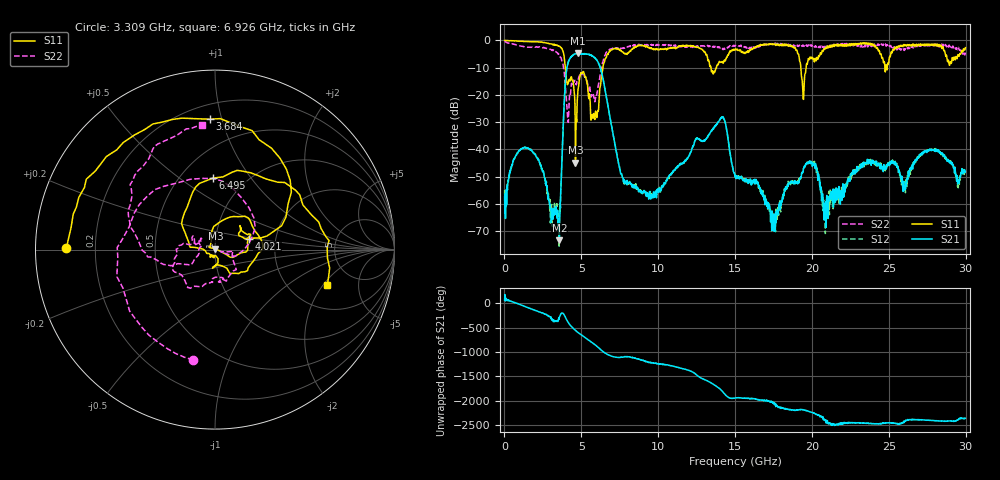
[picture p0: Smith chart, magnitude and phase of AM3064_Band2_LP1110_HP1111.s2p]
# Hz S DB R 50.0
!freq dBS11 angS11 dBS21 angS21 dBS12 angS12 dBS22 angS22
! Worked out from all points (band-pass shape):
!   1600 points, 10 MHz to 29.98 GHz, reference 50 ohm
!   highest |S21| = -4.74 dB at 4.752 GHz (marker M1); lowest = -73.2 dB at 3.571 GHz (marker M2)
!   |S21| within 3 dB of the highest: 4.171 GHz to 6.062 GHz (1.89 GHz wide, 36.9 % of centre)
!   lowest |S11| = -44.8 dB at 4.621 GHz (marker M3), VSWR 1.01, Z = 50.3 + j0.512 ohm
!   |S11| at or under -10 dB: 3.958 GHz to 6.404 GHz (2.446 GHz wide, 47.2 % of centre); 13.43 GHz to 13.78 GHz (351.1 MHz wide, 2.58 % of centre); 19.28 GHz to 19.62 GHz (339.2 MHz wide, 1.74 % of centre)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
!   |S22| runs from -30.1 to -0.2 dB; largest |S21 - S12| = 0.013
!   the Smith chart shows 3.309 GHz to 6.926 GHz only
!   S11 on the Smith chart (normalised r, x): 3.309 GHz: 0.09, +0.01; 3.684 GHz: 0.30, +0.91; 4.021 GHz: 1.45, +0.19; 6.495 GHz: 0.71, +0.67; 6.926 GHz: 3.17, -2.21
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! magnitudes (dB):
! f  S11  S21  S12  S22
! 10 MHz  -0.1  -57.5  -54.9  -0.2
! 1.435 GHz  -0.4  -39.4  -39.4  -2.5
! 3.309 GHz  -1.6  -63.1  -60.8  -4.1
! 3.571 GHz  -2.2  -73.2  -65.6  -5.3
! 3.684 GHz  -2.8  -52.2  -53.5  -6.5
! 4.021 GHz  -14.1  -11.8  -11.7  -21.1
! 4.621 GHz  -44.8  -5.0  -5.0  -15.6
! 4.752 GHz  -20.6  -4.7  -4.7  -14.9
! 5.015 GHz  -12.0  -5.0  -5.0  -12.5
! 5.764 GHz  -27.5  -5.9  -5.8  -20.2
! 6.495 GHz  -8.0  -16.6  -16.6  -6.0
! 6.926 GHz  -3.7  -30.3  -30.2  -3.1
! 7.807 GHz  -4.9  -51.9  -51.5  -2.8
! 10 GHz  -3.4  -54.3  -55.1  -1.8
! 14.14 GHz  -7.8  -28.2  -28.2  -3.0
! 15 GHz  -3.2  -49.9  -49.5  -1.9
! 17.52 GHz  -1.6  -63.7  -64.8  -1.3
! 19.45 GHz  -21.7  -47.0  -47.1  -1.9
! 19.99 GHz  -6.2  -44.9  -45.1  -1.7
! 20.89 GHz  -2.6  -59.1  -59.1  -2.8
! 25 GHz  -8.1  -45.2  -44.7  -1.7
! 29.98 GHz  -2.7  -48.3  -48.8  -4.5
